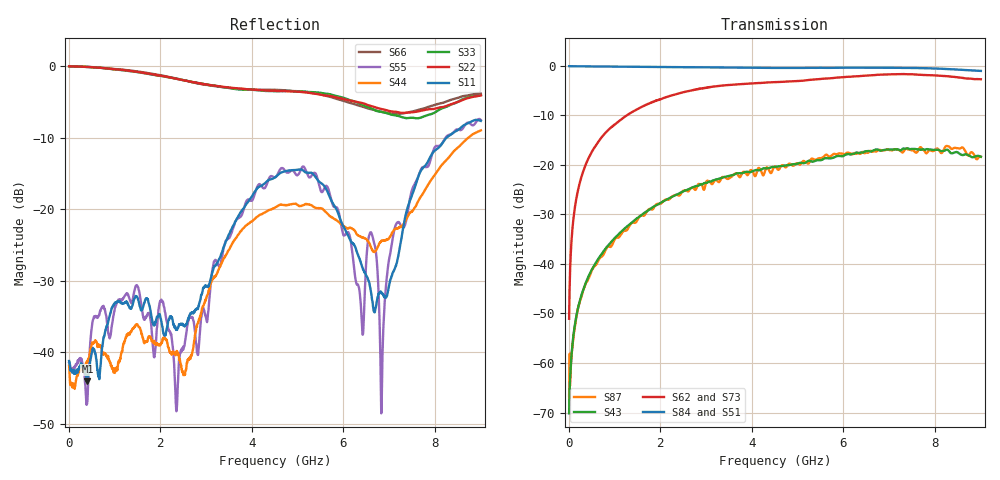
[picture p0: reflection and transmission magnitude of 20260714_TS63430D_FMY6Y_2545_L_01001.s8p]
# GHz S DB R 50
! CMT, SN0916, 25263762, 26.7.0
! Date: 15.07.2026 14:56:17
! Data: Format
! Freq S1.1:dB/Ang S1.2:dB/Ang S1.3:dB/Ang S1.4:dB/Ang S1.5:dB/Ang S1.6:dB/Ang S1.7:dB/Ang S1.8:dB/Ang
!  S2.1:dB/Ang S2.2:dB/Ang S2.3:dB/Ang S2.4:dB/Ang S2.5:dB/Ang S2.6:dB/Ang S2.7:dB/Ang S2.8:dB/Ang
!  S3.1:dB/Ang S3.2:dB/Ang S3.3:dB/Ang S3.4:dB/Ang S3.5:dB/Ang S3.6:dB/Ang S3.7:dB/Ang S3.8:dB/Ang
!  S4.1:dB/Ang S4.2:dB/Ang S4.3:dB/Ang S4.4:dB/Ang S4.5:dB/Ang S4.6:dB/Ang S4.7:dB/Ang S4.8:dB/Ang
!  S5.1:dB/Ang S5.2:dB/Ang S5.3:dB/Ang S5.4:dB/Ang S5.5:dB/Ang S5.6:dB/Ang S5.7:dB/Ang S5.8:dB/Ang
!  S6.1:dB/Ang S6.2:dB/Ang S6.3:dB/Ang S6.4:dB/Ang S6.5:dB/Ang S6.6:dB/Ang S6.7:dB/Ang S6.8:dB/Ang
!  S7.1:dB/Ang S7.2:dB/Ang S7.3:dB/Ang S7.4:dB/Ang S7.5:dB/Ang S7.6:dB/Ang S7.7:dB/Ang S7.8:dB/Ang
!  S8.1:dB/Ang S8.2:dB/Ang S8.3:dB/Ang S8.4:dB/Ang S8.5:dB/Ang S8.6:dB/Ang S8.7:dB/Ang S8.8:dB/Ang
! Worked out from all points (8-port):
!   2001 points, 10 MHz to 9 GHz, reference 50 ohm
!   strongest paths, dB at 10 MHz, 2.257 GHz, 4.505 GHz, 6.753 GHz, 9 GHz:
!     S84: -0.1, -0.3, -0.4, -0.4, -1.0
!     S51: -0.1, -0.2, -0.5, -0.4, -1.3
!     S62: -51.1, -6.0, -3.3, -1.8, -2.7
!     S73: -51.3, -6.1, -3.3, -1.7, -2.8
!     S43: -70.2, -26.4, -20.4, -16.9, -18.4
!     S87: -66.6, -26.4, -20.3, -17.0, -18.3
!   lowest |S11| = -44.1 dB at 410.1 MHz (marker M1), VSWR 1.01, Z = 50.3 - j0.573 ohm
!   |S11| at or under -10 dB: start of sweep to 8.25 GHz
